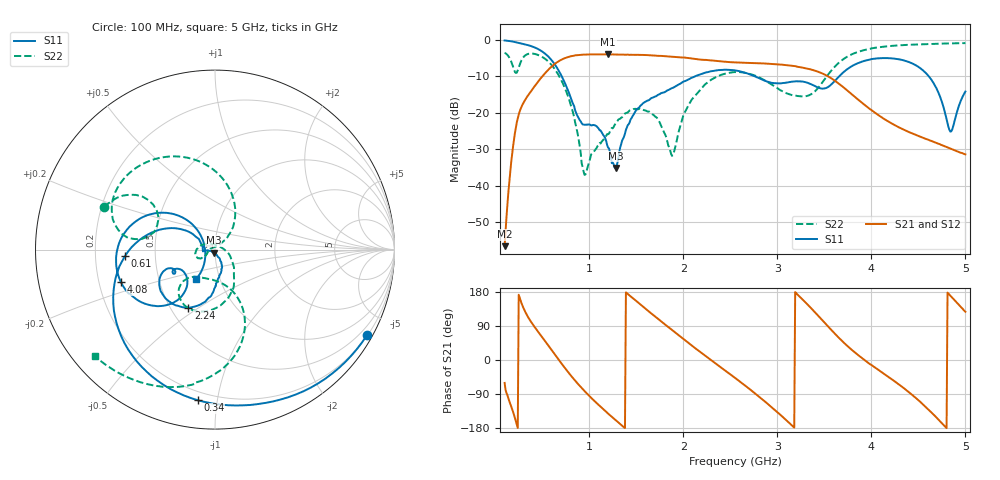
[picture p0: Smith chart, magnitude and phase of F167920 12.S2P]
!  2-Port S-parameters saved by WinCal
! VAR MeasName=S-Parameters (CALIBRATED_DATA) read from VNA (N5242A)
! VAR MeasDate=2016-11-22 9:54:10
! VAR NAME=F167920 12
! VAR FILENAME=F167920 12.S2P
! VAR DATE=2016-11-22 9:54:10
! VAR PHYS_PORTS=1,2
# Hz S DB R 50
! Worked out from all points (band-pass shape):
!   491 points, 100 MHz to 5 GHz, reference 50 ohm
!   highest |S21| = -4.03 dB at 1.2 GHz (marker M1); lowest = -56.5 dB at 100 MHz (marker M2)
!   |S21| within 3 dB of the highest: 615.6 MHz to 3.114 GHz (2.498 GHz wide, 134 % of centre)
!   lowest |S11| = -35.1 dB at 1.28 GHz (marker M3), VSWR 1.04, Z = 49.3 - j1.61 ohm
!   |S11| at or under -10 dB: 706.6 MHz to 2.13 GHz (1.423 GHz wide, 100 % of centre); 2.756 GHz to 3.66 GHz (903.9 MHz wide, 28.2 % of centre); 4.609 GHz to end of sweep
!   |S22| runs from -37.0 to -1.0 dB; largest |S21 - S12| = 0.00098
!   S11 on the Smith chart (normalised r, x): 100 MHz: 0.22, -3.82; 340 MHz: 0.15, -0.88; 610 MHz: 0.33, -0.03; 2.24 GHz: 0.61, -0.45; 4.08 GHz: 0.29, -0.15; 5 GHz: 0.77, -0.26
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1e8  -0.25 -29.3  -56.48 -60.5  -56.43 -60.4  -3.61 159.0
2.1e8  -0.68 -60.8  -25.52 -153.2  -25.53 -153.3  -8.88 150.8
3.4e8  -1.46 -96.5  -15.60 117.2  -15.61 117.2  -4.01 155.6
6.1e8  -5.96 -175.8  -7.15 22.9  -7.14 22.9  -7.27 89.1
8e8  -15.66 145.3  -4.60 -39.5  -4.60 -39.5  -17.54 48.2
9.2e8  -22.88 165.1  -4.14 -73.8  -4.14 -73.8  -33.91 60.6
1.2e9  -29.51 -167.3  -4.03 -141.2  -4.03 -141.2  -25.88 -155.6
1.28e9  -35.11 -111.6  -4.10 -158.6  -4.10 -158.6  -22.91 -145.8
1.48e9  -20.12 -66.8  -4.18 159.9  -4.18 159.9  -18.95 -160.7
1.74e9  -15.04 -86.1  -4.45 107.0  -4.45 107.0  -22.25 160.8
1.89e9  -13.19 -91.1  -4.71 77.3  -4.70 77.3  -31.58 55.8
2.02e9  -11.35 -97.6  -4.94 51.8  -4.92 51.8  -19.73 -29.9
2.24e9  -9.00 -114.6  -5.56 10.5  -5.55 10.4  -12.08 -67.5
2.55e9  -8.40 -143.1  -6.24 -47.0  -6.23 -47.1  -8.89 -108.4
3.06e9  -11.88 -150.4  -6.90 -150.9  -6.89 -150.9  -14.22 -128.9
3.37e9  -12.35 -153.7  -8.27 133.9  -8.26 133.9  -14.79 -82.8
3.68e9  -9.48 -125.9  -12.57 52.2  -12.54 52.1  -5.80 -72.2
4.08e9  -5.12 -161.1  -20.75 -27.1  -20.74 -27.1  -2.10 -103.7
4.19e9  -5.10 -172.3  -22.55 -46.0  -22.57 -46.2  -1.79 -109.9
4.6e9  -9.72 141.6  -27.33 -129.0  -27.34 -129.0  -1.22 -126.9
4.84e9  -25.15 -179.5  -29.81 169.6  -29.84 169.8  -1.05 -134.1
5e9  -14.21 -122.6  -31.40 127.3  -31.40 127.1  -0.98 -138.3
